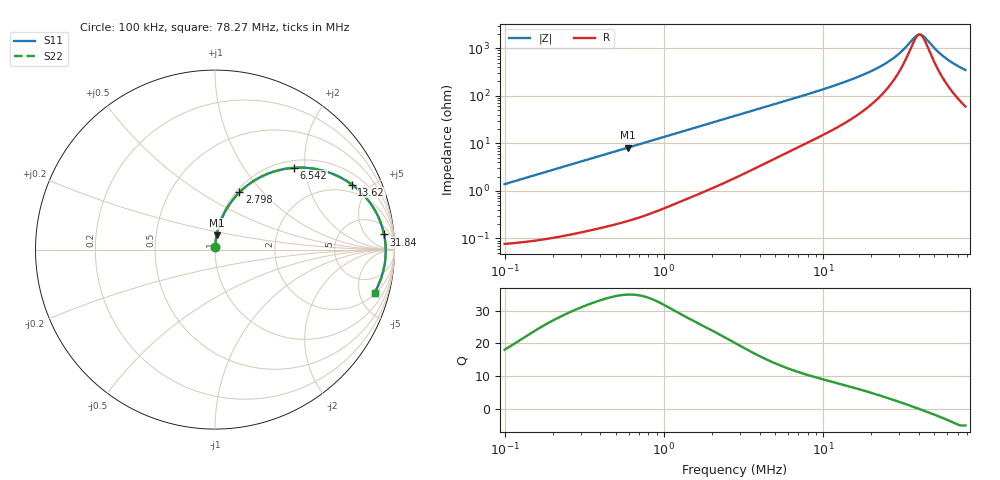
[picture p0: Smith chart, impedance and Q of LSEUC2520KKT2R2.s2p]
! LSEUC2520KKT2R2  S-PARAMETER MODEL  ( General Type )
! Model Generated by TAIYO YUDEN Corporation (http://www.ty-top.com)
! Version 1.0
! TAIYO YUDEN Control No. 220210
! Copyright(c) 2022 TAIYO YUDEN CO.,LTD. All Rights Reserved.
! Product Description (link to TY-COMPAS)
! https://ds.yuden.co.jp/TYCOMPAS/or/detail?pn=LSEUC2520KKT2R2M&u=M
! Products Name : Inductors
! Characteristics :
!  Inductance : 2.2 uH , SRF(min) : -Hz , DC Resistance(max) : 0.076 Ohm
!  Rated Current : Saturation :3000 mA , Temp Rise : 2500 mA (40 degC)
!  Case Size : 2.5 x 2.0 / 0.098 x 0.079 [mm/inch] , Thickness : 1 / 0.039 [mm/inch]
!  (Conditions: Temperature = 25 degC , DC Bias Current/Voltage = 0A / 0V)
! External Node Assignments :
!  1  o---GGG---o  2
! GND o---------o GND
! Frequency Range : 0.1MHz  -  78.268192MHz  [ 402 STEP ]
# MHz S RI R 50
! Freq[MHz].  S11 Real  S11 Imag  S21 Real  S21 Imag  S12 Real  S12 Imag  S22 Real  S22 Imag
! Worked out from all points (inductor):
!   401 points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, 100 kHz to 78.27 MHz, reference 50 ohm
!   read as one part in series: L = 2.2 uH near 103.4 kHz
!   highest Q = 34.9 at 594.3 kHz (marker M1), where L = 2.17 uH
!   self-resonance near 40.32 MHz
!   S11 on the Smith chart (normalised r, x): 100 kHz: 1.00, +0.03; 2.798 MHz: 1.04, +0.75; 6.542 MHz: 1.15, +1.75; 13.62 MHz: 1.53, +3.86; 31.84 MHz: 10, +16; 78.27 MHz: 2.19, -6.87
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0.1  0.000958 0.0138  0.999 -0.0138  0.999 -0.0138  0.000958 0.0138
0.305264  0.0031 0.0418  0.9969 -0.0418  0.9969 -0.0418  0.0031 0.0418
0.594339  0.00882 0.0803  0.9912 -0.0803  0.9912 -0.0803  0.00882 0.0803
0.931861  0.0195 0.1239  0.9805 -0.1239  0.9805 -0.1239  0.0195 0.1239
1.725869  0.0593 0.2174  0.9407 -0.2174  0.9407 -0.2174  0.0593 0.2174
2.797645  0.1361 0.319  0.8639 -0.319  0.8639 -0.319  0.1361 0.319
2.844635  0.1399 0.3227  0.8601 -0.3227  0.8601 -0.3227  0.1399 0.3227
4.242694  0.2583 0.4067  0.7417 -0.4067  0.7417 -0.4067  0.2583 0.4067
6.542214  0.441 0.4558  0.559 -0.4558  0.559 -0.4558  0.441 0.4558
8.540203  0.566 0.4481  0.434 -0.4481  0.434 -0.4481  0.566 0.4481
13.61505  0.7623 0.3626  0.2377 -0.3626  0.2377 -0.3626  0.7623 0.3626
19.64112  0.8703 0.2517  0.1297 -0.2517  0.1297 -0.2517  0.8703 0.2517
26.07016  0.9215 0.1547  0.0785 -0.1547  0.0785 -0.1547  0.9215 0.1547
31.8384  0.942 0.0842  0.058 -0.0842  0.058 -0.0842  0.942 0.0842
37.60892  0.9502 0.0249  0.0498 -0.0249  0.0498 -0.0249  0.9502 0.0249
39.53601  0.9511 0.00702  0.0489 -0.00702  0.0489 -0.00702  0.9511 0.00702
40.87528  0.9513 -0.0049  0.0487 0.0049  0.0487 0.0049  0.9513 -0.0049
43.69146  0.9508 -0.0288  0.0492 0.0288  0.0492 0.0288  0.9508 -0.0288
50.75774  0.9451 -0.0828  0.0549 0.0828  0.0549 0.0828  0.9451 -0.0828
57.99278  0.9344 -0.1311  0.0656 0.1311  0.0656 0.1311  0.9344 -0.1311
67.37203  0.9156 -0.1855  0.0844 0.1855  0.0844 0.1855  0.9156 -0.1855
78.26819  0.8888 -0.2396  0.1112 0.2396  0.1112 0.2396  0.8888 -0.2396
